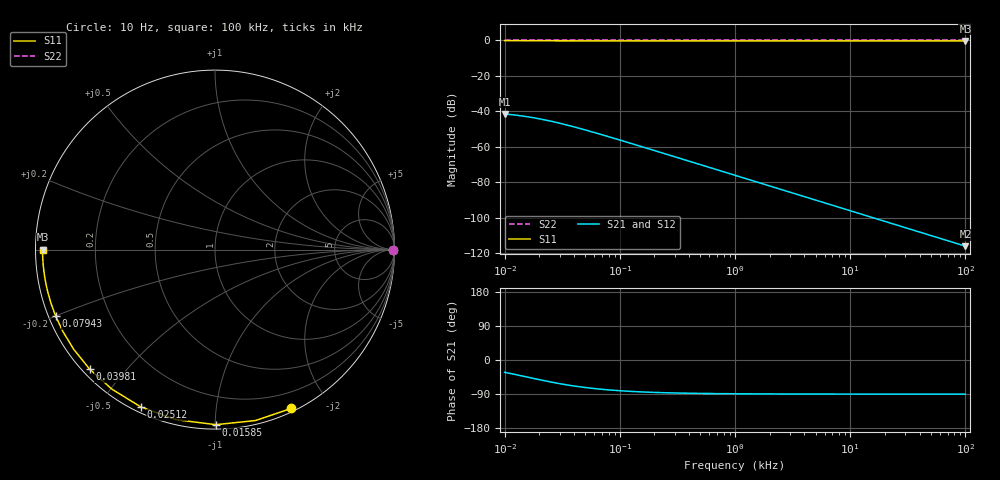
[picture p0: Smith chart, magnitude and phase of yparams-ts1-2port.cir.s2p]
# Hz Y RI R 50
!  Freq  ReY11  ImY11  ReY21  ImY21  ReY12  ImY12  ReY22  ImY22
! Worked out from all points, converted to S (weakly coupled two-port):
!   41 points, 10 Hz to 100 kHz, reference 50 ohm
!   highest |S21| = -41.57 dB at 10 Hz (marker M1); lowest = -116.2 dB at 100 kHz (marker M2)
!   lowest |S11| = -0.3 dB at 100 kHz (marker M3), VSWR 50.00, Z = 1 - j0.00796 ohm
!   |S11| at or under -10 dB: nowhere
!   |S22| runs from -0.1 to -0.1 dB; largest |S21 - S12| = 1.2e-18
!   S11 on the Smith chart (normalised r, x): 10 Hz: 0.03, -1.59; 15.85 Hz: 0.03, -1.00; 25.12 Hz: 0.02, -0.63; 39.81 Hz: 0.02, -0.40; 79.43 Hz: 0.02, -0.20; 100 kHz: 0.02, -0.00
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10  0.0129 0.6281  -0.005 6.28e-05  -0.005 6.28e-05  0.005 6.53e-09
12.58925  0.0175 0.7907  -0.005 7.91e-05  -0.005 7.91e-05  0.005 8.22e-09
15.84893  0.0248 0.9952  -0.005 9.95e-05  -0.005 9.95e-05  0.005 1.03e-08
19.95262  0.0364 1.253  -0.005 0.000125  -0.005 0.000125  0.005 1.3e-08
25.11886  0.0548 1.576  -0.00499 0.000158  -0.00499 0.000158  0.005 1.64e-08
31.62278  0.0838 1.983  -0.00499 0.000198  -0.00499 0.000198  0.005 2.06e-08
39.81072  0.1298 2.495  -0.00499 0.000249  -0.00499 0.000249  0.005 2.59e-08
50.11872  0.2025 3.136  -0.00498 0.000314  -0.00498 0.000314  0.005 3.26e-08
63.09573  0.3173 3.939  -0.00497 0.000394  -0.00497 0.000394  0.005 4.1e-08
79.43282  0.4981 4.941  -0.00495 0.000494  -0.00495 0.000494  0.005 5.14e-08
100  0.7821 6.184  -0.00492 0.000618  -0.00492 0.000618  0.005 6.43e-08
125.8925  1.225 7.715  -0.00488 0.000772  -0.00488 0.000772  0.005 8.03e-08
158.4893  1.912 9.576  -0.00481 0.000958  -0.00481 0.000958  0.005 9.97e-08
251.1886  4.534 14.35  -0.00455 0.00144  -0.00455 0.00144  0.005 1.5e-07
316.2278  6.822 17.16  -0.00432 0.00172  -0.00432 0.00172  0.005 1.79e-07
501.1872  14.2 22.54  -0.00358 0.00225  -0.00358 0.00225  0.005 2.38e-07
794.3282  24.95 25  -0.0025 0.0025  -0.0025 0.0025  0.005 2.7e-07
1258.925  35.72 22.58  -0.00143 0.00226  -0.00143 0.00226  0.005 2.57e-07
1584.893  39.93 20.05  -0.00101 0.002  -0.00101 0.002  0.005 2.4e-07
5011.872  48.77 7.744  -0.000123 0.000774  -0.000123 0.000774  0.005 2.02e-07
25118.86  49.95 1.582  -5.01e-06 0.000158  -5.01e-06 0.000158  0.005 6.39e-07
100000  50 0.3979  -3.09e-07 3.98e-05  -3.09e-07 3.98e-05  0.005 2.49e-06
